PROGRAM P_Prog2
VAR

	fbKL6401 					: FB_LON_KL6401;

	fbREAD_032		: FB_READ_032_SNVT_res_kilo;
	fbSEND_032		: FB_SEND_032_SNVT_res_kilo;

	fbREAD_033		: FB_READ_033_SNVT_sound_db;
	fbSEND_033		: FB_SEND_033_SNVT_sound_db;

	fbREAD_034		: FB_READ_034_SNVT_speed;
	fbSEND_034		: FB_SEND_034_SNVT_speed;

	fbREAD_035		: FB_READ_035_SNVT_speed_mil;
	fbSEND_035		: FB_SEND_035_SNVT_speed_mil;

	fbREAD_036		: FB_READ_036_SNVT_str_asc;
	fbSEND_036		: FB_SEND_036_SNVT_str_asc;

	fbREAD_037		: FB_READ_037_SNVT_str_int;
	fbSEND_037		: FB_SEND_037_SNVT_str_int;

	fbREAD_038		: FB_READ_038_SNVT_telcom;
	fbSEND_038		: FB_SEND_038_SNVT_telcom;

	fbREAD_039		: FB_READ_039_SNVT_temp;
	fbSEND_039		: FB_SEND_039_SNVT_temp;
(*
	fbREAD_040		: FB_READ_040;
	fbSEND_040		: FB_SEND_008_SNVT_count;
*)
	fbREAD_041		: FB_READ_041_SNVT_vol;
	fbSEND_041		: FB_SEND_041_SNVT_vol;

	fbREAD_042		: FB_READ_042_SNVT_vol_kilo;
	fbSEND_042		: FB_SEND_042_SNVT_vol_kilo;

	fbREAD_043		: FB_READ_043_SNVT_vol_mil;
	fbSEND_043		: FB_SEND_043_SNVT_vol_mil;

	fbREAD_044		: FB_READ_044_SNVT_volt;
	fbSEND_044		: FB_SEND_044_SNVT_volt;

	fbREAD_045		: FB_READ_045_SNVT_volt_dbmv;
	fbSEND_045		: FB_SEND_045_SNVT_volt_dbmv;

	fbREAD_046		: FB_READ_046_SNVT_volt_kilo;
	fbSEND_046		: FB_SEND_046_SNVT_volt_kilo;

	fbREAD_047		: FB_READ_047_SNVT_volt_mil;
	fbSEND_047		: FB_SEND_047_SNVT_volt_mil;

	fbREAD_048		: FB_READ_048_SNVT_amp_f;
	fbSEND_048		: FB_SEND_048_SNVT_amp_f;

	fbREAD_049		: FB_READ_049_SNVT_angle_f;
	fbSEND_049		: FB_SEND_049_SNVT_angle_f;

	fbREAD_050		: FB_READ_050_SNVT_angle_vel_f;
	fbSEND_050		: FB_SEND_050_SNVT_angle_vel_f;

	fbREAD_051		: FB_READ_051_SNVT_count_f;
	fbSEND_051		: FB_SEND_051_SNVT_count_f;

	fbREAD_052		: FB_READ_052_SNVT_count_inc_f;
	fbSEND_052		: FB_SEND_052_SNVT_count_inc_f;

	fbREAD_053		: FB_READ_053_SNVT_flow_f;
	fbSEND_053		: FB_SEND_053_SNVT_flow_f;

	fbREAD_054		: FB_READ_054_SNVT_length_f;
	fbSEND_054		: FB_SEND_054_SNVT_length_f;

	fbREAD_055		: FB_READ_055_SNVT_lev_cont_f;
	fbSEND_055		: FB_SEND_055_SNVT_lev_cont_f;

	fbREAD_056		: FB_READ_056_SNVT_mass_f;
	fbSEND_056		: FB_SEND_056_SNVT_mass_f;

	fbREAD_057		: FB_READ_057_SNVT_power_f;
	fbSEND_057		: FB_SEND_057_SNVT_power_f;

	fbREAD_058		: FB_READ_058_SNVT_ppm_f;
	fbSEND_058		: FB_SEND_058_SNVT_ppm_f;

	fbREAD_059		: FB_READ_059_SNVT_press_f;
	fbSEND_059		: FB_SEND_059_SNVT_press_f;

	fbREAD_060		: FB_READ_060_SNVT_res_f;
	fbSEND_060		: FB_SEND_060_SNVT_res_f;

	fbREAD_061		: FB_READ_061_SNVT_sound_db_f;
	fbSEND_061		: FB_SEND_061_SNVT_sound_db_f;

	fbREAD_062		: FB_READ_062_SNVT_speed_f;
	fbSEND_062		: FB_SEND_062_SNVT_speed_f;

END_VAR


fbKL6401(
	bDisabled:=FALSE ,
	stParameter_IN:=LON_IN_2 ,
	stParameter_OUT:=LON_OUT_2 ,
	stLON_Com:=stLON_Com_2,
	bReady=> ,
	eError=> ,
	stKL6401=> ,
	arrProgID=> ,
	arrNeuronID=> ,
	bBusy=> ,
	bError=> ,
	dwErrorKL=> ,
	bTimeOut=> ,
	byLONState=> );

(**)
fbREAD_032(
	wNVIndex:=0 ,
	bDisabled:= ,
	stLON_Com:=stLON_Com_2,
	rValue=> ,
	bNewData=> ,
	bError=> ,
	eError=> );
fbREAD_032.rValue;
fbREAD_032.bError;
fbREAD_032.eError;

fbSEND_032.rValue;
fbSEND_032.bStart;
fbSEND_032.bError;
fbSEND_032.eError;
fbSEND_032.bBusy;
fbSEND_032.dwErrorKL;

fbSEND_032.bAuto;
fbSEND_032.bSendInit;
fbSEND_032.tMinSendTime;
fbSEND_032.tMaxSendTime;
fbSEND_032.rValueLimit;

fbSEND_032(
	wNVIndex:=1 ,
	bStart:= ,
	rValue:= ,
	bDisabled:= ,
	stLON_Com:=stLON_Com_2,
	bError=> ,
	eError=> );
fbSEND_032.bStart:=FALSE;

(**)
fbREAD_033(
	wNVIndex:=2 ,
	bDisabled:= ,
	stLON_Com:=stLON_Com_2,
	rValue=> ,
	bNewData=> ,
	bError=> ,
	eError=> );
fbREAD_033.rValue;
fbREAD_033.bError;
fbREAD_033.eError;

fbSEND_033.rValue;
fbSEND_033.bStart;
fbSEND_033.bError;
fbSEND_033.eError;
fbSEND_033.bBusy;
fbSEND_033.dwErrorKL;

fbSEND_033.bAuto;
fbSEND_033.bSendInit;
fbSEND_033.tMinSendTime;
fbSEND_033.tMaxSendTime;
fbSEND_033.rValueLimit;

fbSEND_033(
	wNVIndex:=3 ,
	bStart:= ,
	rValue:= ,
	bDisabled:= ,
	stLON_Com:=stLON_Com_2,
	bError=> ,
	eError=> );
fbSEND_033.bStart:=FALSE;

(**)
fbREAD_034(
	wNVIndex:=4 ,
	bDisabled:= ,
	stLON_Com:=stLON_Com_2,
	rValue=> ,
	bNewData=> ,
	bError=> ,
	eError=> );
fbREAD_034.rValue;
fbREAD_034.bError;
fbREAD_034.eError;

fbSEND_034.rValue;
fbSEND_034.bStart;
fbSEND_034.bError;
fbSEND_034.eError;
fbSEND_034.bBusy;
fbSEND_034.dwErrorKL;

fbSEND_034.bAuto;
fbSEND_034.bSendInit;
fbSEND_034.tMinSendTime;
fbSEND_034.tMaxSendTime;
fbSEND_034.rValueLimit;

fbSEND_034(
	wNVIndex:=5 ,
	bStart:= ,
	rValue:= ,
	bDisabled:= ,
	stLON_Com:=stLON_Com_2,
	bError=> ,
	eError=> );
fbSEND_034.bStart:=FALSE;

(**)
fbREAD_035(
	wNVIndex:=6 ,
	bDisabled:= ,
	stLON_Com:=stLON_Com_2,
	rValue=> ,
	bNewData=> ,
	bError=> ,
	eError=> );
fbREAD_035.rValue;
fbREAD_035.bError;
fbREAD_035.eError;

fbSEND_035.rValue;
fbSEND_035.bStart;
fbSEND_035.bError;
fbSEND_035.eError;
fbSEND_035.bBusy;
fbSEND_035.dwErrorKL;

fbSEND_035.bAuto;
fbSEND_035.bSendInit;
fbSEND_035.tMinSendTime;
fbSEND_035.tMaxSendTime;
fbSEND_035.rValueLimit;

fbSEND_035(
	wNVIndex:=7 ,
	bStart:= ,
	rValue:= ,
	bDisabled:= ,
	stLON_Com:=stLON_Com_2,
	bError=> ,
	eError=> );
fbSEND_035.bStart:=FALSE;

(**)
fbREAD_036(
	wNVIndex:=8 ,
	bDisabled:= ,
	stLON_Com:=stLON_Com_2,
	sValue=> ,
	bNewData=> ,
	bError=> ,
	eError=> );
fbREAD_036.sValue;
fbREAD_036.bError;
fbREAD_036.eError;

fbSEND_036.sValue;
fbSEND_036.bStart;
fbSEND_036.bError;
fbSEND_036.eError;
fbSEND_036.bBusy;
fbSEND_036.dwErrorKL;

fbSEND_036.bAuto;
fbSEND_036.bSendInit;
fbSEND_036.tMinSendTime;
fbSEND_036.tMaxSendTime;

fbSEND_036(
	wNVIndex:=9 ,
	bStart:= ,
	sValue:= ,
	bDisabled:= ,
	stLON_Com:=stLON_Com_2,
	bError=> ,
	eError=> );
fbSEND_036.bStart:=FALSE;

(**)
fbREAD_037(
	wNVIndex:=10 ,
	bDisabled:= ,
	stLON_Com:=stLON_Com_2,
	stValue=> ,
	bNewData=> ,
	bError=> ,
	eError=> );
fbREAD_037.stValue;
fbREAD_037.bError;
fbREAD_037.eError;

fbSEND_037.stValue;
fbSEND_037.bStart;
fbSEND_037.bError;
fbSEND_037.eError;
fbSEND_037.bBusy;
fbSEND_037.dwErrorKL;

fbSEND_037.bAuto;
fbSEND_037.bSendInit;
fbSEND_037.tMinSendTime;
fbSEND_037.tMaxSendTime;

fbSEND_037(
	wNVIndex:=11 ,
	bStart:= ,
	stValue:= ,
	bDisabled:= ,
	stLON_Com:=stLON_Com_2,
	bError=> ,
	eError=> );
fbSEND_037.bStart:=FALSE;

(**)
fbREAD_038(
	wNVIndex:=12 ,
	bDisabled:= ,
	stLON_Com:=stLON_Com_2,
	eValue=> ,
	bNewData=> ,
	bError=> ,
	eError=> );
fbREAD_038.eValue;
fbREAD_038.bError;
fbREAD_038.eError;

fbSEND_038.eValue;
fbSEND_038.bStart;
fbSEND_038.bError;
fbSEND_038.eError;
fbSEND_038.bBusy;
fbSEND_038.dwErrorKL;

fbSEND_038.bAuto;
fbSEND_038.bSendInit;
fbSEND_038.tMinSendTime;
fbSEND_038.tMaxSendTime;

fbSEND_038(
	wNVIndex:=13 ,
	bStart:= ,
	eValue:= ,
	bDisabled:= ,
	stLON_Com:=stLON_Com_2,
	bError=> ,
	eError=> );
fbSEND_038.bStart:=FALSE;

(**)
fbREAD_039(
	wNVIndex:=14 ,
	bDisabled:= ,
	stLON_Com:=stLON_Com_2,
	rValue=> ,
	bNewData=> ,
	bError=> ,
	eError=> );
fbREAD_039.rValue;
fbREAD_039.bError;
fbREAD_039.eError;

fbSEND_039.rValue;
fbSEND_039.bStart;
fbSEND_039.bError;
fbSEND_039.eError;
fbSEND_039.bBusy;
fbSEND_039.dwErrorKL;

fbSEND_039.bAuto;
fbSEND_039.bSendInit;
fbSEND_039.tMinSendTime;
fbSEND_039.tMaxSendTime;
fbSEND_039.rValueLimit;

fbSEND_039(
	wNVIndex:=15 ,
	bStart:= ,
	rValue:= ,
	bDisabled:= ,
	stLON_Com:=stLON_Com_2,
	bError=> ,
	eError=> );
fbSEND_039.bStart:=FALSE;

(**)
(*
fbREAD_040(
	wNVIndex:=16 ,
	bDisabled:= ,
	stLON_Com:=stLON_Com_2,
	uiValue=> ,
	bNewData=> ,
	bError=> ,
	eError=> );
fbREAD_040.uiValue;
fbREAD_040.bError;
fbREAD_040.eError;

fbSEND_040(
	wNVIndex:=17 ,
	bStart:= ,
	uiValue:= ,
	bDisabled:= ,
	stLON_Com:=stLON_Com_2,
	bError=> ,
	eError=> );
fbSEND_040.uiValue;
fbSEND_040.bStart;
fbSEND_040.bError;
fbSEND_040.eError;
*)

(**)
fbREAD_041(
	wNVIndex:=18 ,
	bDisabled:= ,
	stLON_Com:=stLON_Com_2,
	rValue=> ,
	bNewData=> ,
	bError=> ,
	eError=> );
fbREAD_041.rValue;
fbREAD_041.bError;
fbREAD_041.eError;

fbSEND_041.rValue;
fbSEND_041.bStart;
fbSEND_041.bError;
fbSEND_041.eError;
fbSEND_041.bBusy;
fbSEND_041.dwErrorKL;

fbSEND_041.bAuto;
fbSEND_041.bSendInit;
fbSEND_041.tMinSendTime;
fbSEND_041.tMaxSendTime;
fbSEND_041.rValueLimit;

fbSEND_041(
	wNVIndex:=19 ,
	bStart:= ,
	rValue:= ,
	bDisabled:= ,
	stLON_Com:=stLON_Com_2,
	bError=> ,
	eError=> );
fbSEND_041.bStart:=FALSE;

(**)
fbREAD_042(
	wNVIndex:=20 ,
	bDisabled:= ,
	stLON_Com:=stLON_Com_2,
	rValue=> ,
	bNewData=> ,
	bError=> ,
	eError=> );
fbREAD_042.rValue;
fbREAD_042.bError;
fbREAD_042.eError;

fbSEND_042.rValue;
fbSEND_042.bStart;
fbSEND_042.bError;
fbSEND_042.eError;
fbSEND_042.bBusy;
fbSEND_042.dwErrorKL;

fbSEND_042.bAuto;
fbSEND_042.bSendInit;
fbSEND_042.tMinSendTime;
fbSEND_042.tMaxSendTime;
fbSEND_042.rValueLimit;

fbSEND_042(
	wNVIndex:=21 ,
	bStart:= ,
	rValue:= ,
	bDisabled:= ,
	stLON_Com:=stLON_Com_2,
	bError=> ,
	eError=> );
fbSEND_042.bStart:=FALSE;

(**)
fbREAD_043(
	wNVIndex:=22 ,
	bDisabled:= ,
	stLON_Com:=stLON_Com_2,
	rValue=> ,
	bNewData=> ,
	bError=> ,
	eError=> );
fbREAD_043.rValue;
fbREAD_043.bError;
fbREAD_043.eError;

fbSEND_043.rValue;
fbSEND_043.bStart;
fbSEND_043.bError;
fbSEND_043.eError;
fbSEND_043.bBusy;
fbSEND_043.dwErrorKL;

fbSEND_043.bAuto;
fbSEND_043.bSendInit;
fbSEND_043.tMinSendTime;
fbSEND_043.tMaxSendTime;
fbSEND_043.rValueLimit;

fbSEND_043(
	wNVIndex:=23 ,
	bStart:= ,
	rValue:= ,
	bDisabled:= ,
	stLON_Com:=stLON_Com_2,
	bError=> ,
	eError=> );
fbSEND_043.bStart:=FALSE;

(**)
fbREAD_044(
	wNVIndex:=24 ,
	bDisabled:= ,
	stLON_Com:=stLON_Com_2,
	rValue=> ,
	bNewData=> ,
	bError=> ,
	eError=> );
fbREAD_044.rValue;
fbREAD_044.bError;
fbREAD_044.eError;

fbSEND_044.rValue;
fbSEND_044.bStart;
fbSEND_044.bError;
fbSEND_044.eError;
fbSEND_044.bBusy;
fbSEND_044.dwErrorKL;

fbSEND_044.bAuto;
fbSEND_044.bSendInit;
fbSEND_044.tMinSendTime;
fbSEND_044.tMaxSendTime;
fbSEND_044.rValueLimit;

fbSEND_044(
	wNVIndex:=25 ,
	bStart:= ,
	rValue:= ,
	bDisabled:= ,
	stLON_Com:=stLON_Com_2,
	bError=> ,
	eError=> );
fbSEND_044.bStart:=FALSE;

(**)
fbREAD_045(
	wNVIndex:=26 ,
	bDisabled:= ,
	stLON_Com:=stLON_Com_2,
	rValue=> ,
	bNewData=> ,
	bError=> ,
	eError=> );
fbREAD_045.rValue;
fbREAD_045.bError;
fbREAD_045.eError;

fbSEND_045.rValue;
fbSEND_045.bStart;
fbSEND_045.bError;
fbSEND_045.eError;

fbSEND_045.bAuto;
fbSEND_045.bSendInit;
fbSEND_045.tMinSendTime;
fbSEND_045.tMaxSendTime;
fbSEND_045.rValueLimit;
fbSEND_045.bBusy;
fbSEND_045.dwErrorKL;

fbSEND_045(
	wNVIndex:=27 ,
	bStart:= ,
	rValue:= ,
	bDisabled:= ,
	stLON_Com:=stLON_Com_2,
	bError=> ,
	eError=> );
fbSEND_045.bStart:=FALSE;

(**)
fbREAD_046(
	wNVIndex:=28 ,
	bDisabled:= ,
	stLON_Com:=stLON_Com_2,
	rValue=> ,
	bNewData=> ,
	bError=> ,
	eError=> );
fbREAD_046.rValue;
fbREAD_046.bError;
fbREAD_046.eError;

fbSEND_046.rValue;
fbSEND_046.bStart;
fbSEND_046.bError;
fbSEND_046.eError;
fbSEND_046.bBusy;
fbSEND_046.dwErrorKL;

fbSEND_046.bAuto;
fbSEND_046.bSendInit;
fbSEND_046.tMinSendTime;
fbSEND_046.tMaxSendTime;
fbSEND_046.rValueLimit;

fbSEND_046(
	wNVIndex:=29 ,
	bStart:= ,
	rValue:= ,
	bDisabled:= ,
	stLON_Com:=stLON_Com_2,
	bError=> ,
	eError=> );
fbSEND_046.bStart:=FALSE;


(**)
fbREAD_047(
	wNVIndex:=30 ,
	bDisabled:= ,
	stLON_Com:=stLON_Com_2,
	rValue=> ,
	bNewData=> ,
	bError=> ,
	eError=> );
fbREAD_047.rValue;
fbREAD_047.bError;
fbREAD_047.eError;

fbSEND_047.rValue;
fbSEND_047.bStart;
fbSEND_047.bError;
fbSEND_047.eError;
fbSEND_047.bBusy;
fbSEND_047.dwErrorKL;

fbSEND_047.bAuto;
fbSEND_047.bSendInit;
fbSEND_047.tMinSendTime;
fbSEND_047.tMaxSendTime;
fbSEND_047.rValueLimit;

fbSEND_047(
	wNVIndex:=31 ,
	bStart:= ,
	rValue:= ,
	bDisabled:= ,
	stLON_Com:=stLON_Com_2,
	bError=> ,
	eError=> );
fbSEND_047.bStart:=FALSE;

(**)
fbREAD_048(
	wNVIndex:=32 ,
	bDisabled:= ,
	stLON_Com:=stLON_Com_2,
	rValue=> ,
	bNewData=> ,
	bError=> ,
	eError=> );
fbREAD_048.rValue;
fbREAD_048.bError;
fbREAD_048.eError;

fbSEND_048.rValue;
fbSEND_048.bStart;
fbSEND_048.bError;
fbSEND_048.eError;
fbSEND_048.bBusy;
fbSEND_048.dwErrorKL;

fbSEND_048.bAuto;
fbSEND_048.bSendInit;
fbSEND_048.tMinSendTime;
fbSEND_048.tMaxSendTime;
fbSEND_048.rValueLimit;

fbSEND_048(
	wNVIndex:=33 ,
	bStart:= ,
	rValue:= ,
	bDisabled:= ,
	stLON_Com:=stLON_Com_2,
	bError=> ,
	eError=> );
fbSEND_048.bStart:=FALSE;

(**)
fbREAD_049(
	wNVIndex:=34 ,
	bDisabled:= ,
	stLON_Com:=stLON_Com_2,
	rValue=> ,
	bNewData=> ,
	bError=> ,
	eError=> );
fbREAD_049.rValue;
fbREAD_049.bError;
fbREAD_049.eError;

fbSEND_049.rValue;
fbSEND_049.bStart;
fbSEND_049.bError;
fbSEND_049.eError;
fbSEND_049.bBusy;
fbSEND_049.dwErrorKL;

fbSEND_049.bAuto;
fbSEND_049.bSendInit;
fbSEND_049.tMinSendTime;
fbSEND_049.tMaxSendTime;
fbSEND_049.rValueLimit;

fbSEND_049(
	wNVIndex:=35 ,
	bStart:= ,
	rValue:= ,
	bDisabled:= ,
	stLON_Com:=stLON_Com_2,
	bError=> ,
	eError=> );
fbSEND_049.bStart:=FALSE;

(**)
fbREAD_050(
	wNVIndex:=36 ,
	bDisabled:= ,
	stLON_Com:=stLON_Com_2,
	rValue=> ,
	bNewData=> ,
	bError=> ,
	eError=> );
fbREAD_050.rValue;
fbREAD_050.bError;
fbREAD_050.eError;

fbSEND_050.rValue;
fbSEND_050.bStart;
fbSEND_050.bError;
fbSEND_050.eError;
fbSEND_050.bBusy;
fbSEND_050.dwErrorKL;

fbSEND_050.bAuto;
fbSEND_050.bSendInit;
fbSEND_050.tMinSendTime;
fbSEND_050.tMaxSendTime;
fbSEND_050.rValueLimit;

fbSEND_050(
	wNVIndex:=37 ,
	bStart:= ,
	rValue:= ,
	bDisabled:= ,
	stLON_Com:=stLON_Com_2,
	bError=> ,
	eError=> );
fbSEND_050.bStart:=FALSE;

(**)
fbREAD_051(
	wNVIndex:=38 ,
	bDisabled:= ,
	stLON_Com:=stLON_Com_2,
	rValue=> ,
	bNewData=> ,
	bError=> ,
	eError=> );
fbREAD_051.rValue;
fbREAD_051.bError;
fbREAD_051.eError;

fbSEND_051.rValue;
fbSEND_051.bStart;
fbSEND_051.bError;
fbSEND_051.eError;

fbSEND_051.bAuto;
fbSEND_051.bSendInit;
fbSEND_051.tMinSendTime;
fbSEND_051.tMaxSendTime;
fbSEND_051.rValueLimit;
fbSEND_051.bBusy;
fbSEND_051.dwErrorKL;

fbSEND_051(
	wNVIndex:=39 ,
	bStart:= ,
	rValue:= ,
	bDisabled:= ,
	stLON_Com:=stLON_Com_2,
	bError=> ,
	eError=> );
fbSEND_051.bStart:=FALSE;

(**)
fbREAD_052(
	wNVIndex:=40 ,
	bDisabled:= ,
	stLON_Com:=stLON_Com_2,
	rValue=> ,
	bNewData=> ,
	bError=> ,
	eError=> );
fbREAD_052.rValue;
fbREAD_052.bError;
fbREAD_052.eError;

fbSEND_052.rValue;
fbSEND_052.bStart;
fbSEND_052.bError;
fbSEND_052.eError;
fbSEND_052.bBusy;
fbSEND_052.dwErrorKL;

fbSEND_052.bAuto;
fbSEND_052.bSendInit;
fbSEND_052.tMinSendTime;
fbSEND_052.tMaxSendTime;
fbSEND_052.rValueLimit;

fbSEND_052(
	wNVIndex:=41 ,
	bStart:= ,
	rValue:= ,
	bDisabled:= ,
	stLON_Com:=stLON_Com_2,
	bError=> ,
	eError=> );
fbSEND_052.bStart:=FALSE;

(**)
fbREAD_053(
	wNVIndex:=42 ,
	bDisabled:= ,
	stLON_Com:=stLON_Com_2,
	rValue=> ,
	bNewData=> ,
	bError=> ,
	eError=> );
fbREAD_053.rValue;
fbREAD_053.bError;
fbREAD_053.eError;

fbSEND_053.rValue;
fbSEND_053.bStart;
fbSEND_053.bError;
fbSEND_053.eError;
fbSEND_053.bBusy;
fbSEND_053.dwErrorKL;

fbSEND_053.bAuto;
fbSEND_053.bSendInit;
fbSEND_053.tMinSendTime;
fbSEND_053.tMaxSendTime;
fbSEND_053.rValueLimit;

fbSEND_053(
	wNVIndex:=43 ,
	bStart:= ,
	rValue:= ,
	bDisabled:= ,
	stLON_Com:=stLON_Com_2,
	bError=> ,
	eError=> );
fbSEND_053.bStart:=FALSE;

(**)
fbREAD_054(
	wNVIndex:=44 ,
	bDisabled:= ,
	stLON_Com:=stLON_Com_2,
	rValue=> ,
	bNewData=> ,
	bError=> ,
	eError=> );
fbREAD_054.rValue;
fbREAD_054.bError;
fbREAD_054.eError;

fbSEND_054.rValue;
fbSEND_054.bStart;
fbSEND_054.bError;
fbSEND_054.eError;
fbSEND_054.bBusy;
fbSEND_054.dwErrorKL;

fbSEND_054.bAuto;
fbSEND_054.bSendInit;
fbSEND_054.tMinSendTime;
fbSEND_054.tMaxSendTime;
fbSEND_054.rValueLimit;

fbSEND_054(
	wNVIndex:=45 ,
	bStart:= ,
	rValue:= ,
	bDisabled:= ,
	stLON_Com:=stLON_Com_2,
	bError=> ,
	eError=> );
fbSEND_054.bStart:=FALSE;

(**)
fbREAD_055(
	wNVIndex:=46 ,
	bDisabled:= ,
	stLON_Com:=stLON_Com_2,
	rValue=> ,
	bNewData=> ,
	bError=> ,
	eError=> );
fbREAD_055.rValue;
fbREAD_055.bError;
fbREAD_055.eError;

fbSEND_055.rValue;
fbSEND_055.bStart;
fbSEND_055.bError;
fbSEND_055.eError;
fbSEND_055.bBusy;
fbSEND_055.dwErrorKL;

fbSEND_055.bAuto;
fbSEND_055.bSendInit;
fbSEND_055.tMinSendTime;
fbSEND_055.tMaxSendTime;
fbSEND_055.rValueLimit;

fbSEND_055(
	wNVIndex:=47 ,
	bStart:= ,
	rValue:= ,
	bDisabled:= ,
	stLON_Com:=stLON_Com_2,
	bError=> ,
	eError=> );
fbSEND_055.bStart:=FALSE;

(**)
fbREAD_056(
	wNVIndex:=48 ,
	bDisabled:= ,
	stLON_Com:=stLON_Com_2,
	rValue=> ,
	bNewData=> ,
	bError=> ,
	eError=> );
fbREAD_056.rValue;
fbREAD_056.bError;
fbREAD_056.eError;

fbSEND_056.rValue;
fbSEND_056.bStart;
fbSEND_056.bError;
fbSEND_056.eError;
fbSEND_056.bBusy;
fbSEND_056.dwErrorKL;

fbSEND_056.bAuto;
fbSEND_056.bSendInit;
fbSEND_056.tMinSendTime;
fbSEND_056.tMaxSendTime;
fbSEND_056.rValueLimit;

fbSEND_056(
	wNVIndex:=49 ,
	bStart:= ,
	rValue:= ,
	bDisabled:= ,
	stLON_Com:=stLON_Com_2,
	bError=> ,
	eError=> );
fbSEND_056.bStart:=FALSE;

(**)
fbREAD_057(
	wNVIndex:=50 ,
	bDisabled:= ,
	stLON_Com:=stLON_Com_2,
	rValue=> ,
	bNewData=> ,
	bError=> ,
	eError=> );
fbREAD_057.rValue;
fbREAD_057.bError;
fbREAD_057.eError;

fbSEND_057.rValue;
fbSEND_057.bStart;
fbSEND_057.bError;
fbSEND_057.eError;
fbSEND_057.bBusy;
fbSEND_057.dwErrorKL;

fbSEND_057.bAuto;
fbSEND_057.bSendInit;
fbSEND_057.tMinSendTime;
fbSEND_057.tMaxSendTime;
fbSEND_057.rValueLimit;

fbSEND_057(
	wNVIndex:=51 ,
	bStart:= ,
	rValue:= ,
	bDisabled:= ,
	stLON_Com:=stLON_Com_2,
	bError=> ,
	eError=> );
fbSEND_057.bStart:=FALSE;

(**)
fbREAD_058(
	wNVIndex:=52 ,
	bDisabled:= ,
	stLON_Com:=stLON_Com_2,
	rValue=> ,
	bNewData=> ,
	bError=> ,
	eError=> );
fbREAD_058.rValue;
fbREAD_058.bError;
fbREAD_058.eError;

fbSEND_058.rValue;
fbSEND_058.bStart;
fbSEND_058.bError;
fbSEND_058.eError;
fbSEND_058.bBusy;
fbSEND_058.dwErrorKL;

fbSEND_058.bAuto;
fbSEND_058.bSendInit;
fbSEND_058.tMinSendTime;
fbSEND_058.tMaxSendTime;
fbSEND_058.rValueLimit;

fbSEND_058(
	wNVIndex:=53 ,
	bStart:= ,
	rValue:= ,
	bDisabled:= ,
	stLON_Com:=stLON_Com_2,
	bError=> ,
	eError=> );
fbSEND_058.bStart:=FALSE;

(**)
fbREAD_059(
	wNVIndex:=54 ,
	bDisabled:= ,
	stLON_Com:=stLON_Com_2,
	rValue=> ,
	bNewData=> ,
	bError=> ,
	eError=> );
fbREAD_059.rValue;
fbREAD_059.bError;
fbREAD_059.eError;

fbSEND_059.rValue;
fbSEND_059.bStart;
fbSEND_059.bError;
fbSEND_059.eError;
fbSEND_059.bBusy;
fbSEND_059.dwErrorKL;

fbSEND_059.bAuto;
fbSEND_059.bSendInit;
fbSEND_059.tMinSendTime;
fbSEND_059.tMaxSendTime;
fbSEND_059.rValueLimit;

fbSEND_059(
	wNVIndex:=55 ,
	bStart:= ,
	rValue:= ,
	bDisabled:= ,
	stLON_Com:=stLON_Com_2,
	bError=> ,
	eError=> );
fbSEND_059.bStart:=FALSE;

(**)
fbREAD_060(
	wNVIndex:=56 ,
	bDisabled:= ,
	stLON_Com:=stLON_Com_2,
	rValue=> ,
	bNewData=> ,
	bError=> ,
	eError=> );
fbREAD_060.rValue;
fbREAD_060.bError;
fbREAD_060.eError;

fbSEND_060.rValue;
fbSEND_060.bStart;
fbSEND_060.bError;
fbSEND_060.eError;
fbSEND_060.bBusy;
fbSEND_060.dwErrorKL;

fbSEND_060.bAuto;
fbSEND_060.bSendInit;
fbSEND_060.tMinSendTime;
fbSEND_060.tMaxSendTime;
fbSEND_060.rValueLimit;

fbSEND_060(
	wNVIndex:=57 ,
	bStart:= ,
	rValue:= ,
	bDisabled:= ,
	stLON_Com:=stLON_Com_2,
	bError=> ,
	eError=> );
fbSEND_060.bStart:=FALSE;

(**)
fbREAD_061(
	wNVIndex:=58 ,
	bDisabled:= ,
	stLON_Com:=stLON_Com_2,
	rValue=> ,
	bNewData=> ,
	bError=> ,
	eError=> );
fbREAD_061.rValue;
fbREAD_061.bError;
fbREAD_061.eError;

fbSEND_061.rValue;
fbSEND_061.bStart;
fbSEND_061.bError;
fbSEND_061.eError;
fbSEND_061.bBusy;
fbSEND_061.dwErrorKL;

fbSEND_061.bAuto;
fbSEND_061.bSendInit;
fbSEND_061.tMinSendTime;
fbSEND_061.tMaxSendTime;
fbSEND_061.rValueLimit;

fbSEND_061(
	wNVIndex:=59 ,
	bStart:= ,
	rValue:= ,
	bDisabled:= ,
	stLON_Com:=stLON_Com_2,
	bError=> ,
	eError=> );
fbSEND_061.bStart:=FALSE;

(**)
fbREAD_062(
	wNVIndex:=60 ,
	bDisabled:= ,
	stLON_Com:=stLON_Com_2,
	rValue=> ,
	bNewData=> ,
	bError=> ,
	eError=> );
fbREAD_062.rValue;
fbREAD_062.bError;
fbREAD_062.eError;

fbSEND_062.rValue;
fbSEND_062.bStart;
fbSEND_062.bError;
fbSEND_062.eError;
fbSEND_062.bBusy;
fbSEND_062.dwErrorKL;

fbSEND_062.bAuto;
fbSEND_062.bSendInit;
fbSEND_062.tMinSendTime;
fbSEND_062.tMaxSendTime;
fbSEND_062.rValueLimit;

fbSEND_062(
	wNVIndex:=61 ,
	bStart:= ,
	rValue:= ,
	bDisabled:= ,
	stLON_Com:=stLON_Com_2,
	bError=> ,
	eError=> );
fbSEND_062.bStart:=FALSE;

END_PROGRAM
